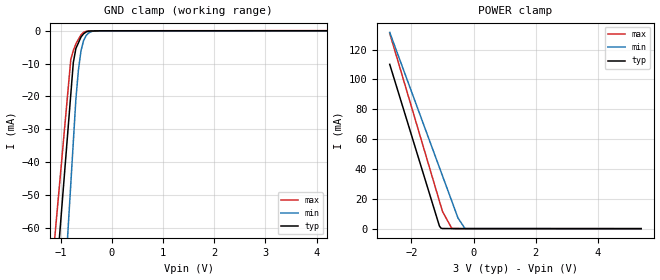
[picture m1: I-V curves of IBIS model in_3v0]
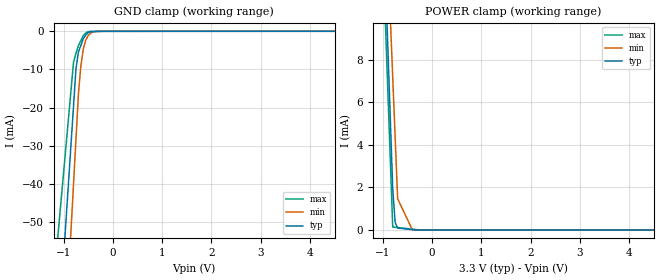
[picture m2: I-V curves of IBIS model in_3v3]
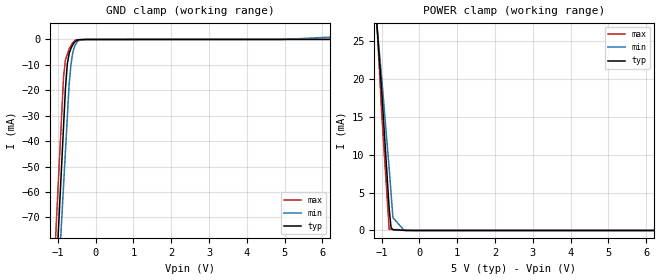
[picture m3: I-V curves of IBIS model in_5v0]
[IBIS Ver]   3.2
[Comment Char] |_char
[File Name]   tlv2553ipw.ibs
[File Rev]   3.0
[Source]
| This model file was created by Teraspeed Consulting Group LLC
| (http://www.teraspeed.com/).
[Date]   09-13-2007
[Notes]   Quality Check of this IBIS model: Model Passes IBIS Check
   Model parses into ICX IS. Simulation done with Hyperlynx.
   1. MIN TYP MAX information is based on Temprature and Voltage
   characteristics only.
[Disclaimer]
| This model is designed as an aid for customers of Texas Instruments.
| TI and its licensors and suppliers make no warranties, either expressed
| or implied, with respect to this  model, including the warranties of
| merchantability or fitness for a particular purpose.
| The model is provided solely on an "as is" basis. The entire risk as to
| its quality and performance is with the customer.
[Copyright]
| (C) Copyright 2008 Texas Instruments Incorporated. All rights reserved.
[Component] TLV2553IPW
[Manufacturer] TI
[Package]
| variable   typ   min   max
R_pkg  1.7363E-02  1.7363E-02  1.7363E-02
L_pkg  2.1878E-09  2.1878E-09  2.1878E-09
C_pkg  4.4649E-13  4.4649E-13  4.4649E-13
[Pin] signal_name  model_name  R_pin  L_pin C_pin
1   AIN0   term   1.97E-02  2.49E-09  5.07E-13
2   AIN1   term   1.89E-02  2.38E-09  4.85E-13
3   AIN2   term   1.80E-02  2.27E-09  4.64E-13
4   AIN3   term   1.72E-02  2.17E-09  4.42E-13
5   AIN4   term   1.64E-02  2.07E-09  4.22E-13
6   AIN5   term   1.56E-02  1.97E-09  4.02E-13
7   AIN6   term   1.49E-02  1.87E-09  3.82E-13
8   AIN7   term   1.49E-02  1.87E-09  3.82E-13
9   AIN8   term   1.56E-02  1.97E-09  4.02E-13
10   GND   GND   1.64E-02  2.07E-09  4.22E-13
11   AIN9   term   1.72E-02  2.17E-09  4.42E-13
12   AIN10   term   1.80E-02  2.27E-09  4.64E-13
13   REF-   term   1.89E-02  2.38E-09  4.85E-13
14   REF+   term   1.97E-02  2.49E-09  5.07E-13
15   _CS   input   1.97E-02  2.49E-09  5.07E-13
16   DATA_OUT  tri   1.89E-02  2.38E-09  4.85E-13
17   DATA_IN   input   1.80E-02  2.27E-09  4.64E-13
18   I/O_CLOCK input   1.72E-02  2.17E-09  4.42E-13
19   EOC   out   1.64E-02  2.07E-09  4.22E-13
20   VCC   POWER   1.56E-02  1.97E-09  4.02E-13
[Model Selector] input
in_3v0  3.0v input
in_3v3  3.3v input
in_5v0  5.0v input
[Model Selector] out
out_3v0  3.0v output
out_3v3  3.3v output
out_5v0  5.0v output
[Model Selector] tri
tri_3v0  3.0v 3-state
tri_3v3  3.3v 3-state
tri_5v0  5.0v 3-state
[Model] term
Model_type Terminator
C_comp  0pF 0pF 0pF
| variable typ   min   max
[Voltage Range]   5.00000V  4.50000V  5.50000V
[POWER Clamp Reference]  5.00000V  4.50000V  5.50000V
[GND Clamp Reference]   0.00000V  0.00000V  0.00000V
[Temperature Range]   25   105   -40
| Models and submodels in the file (10): in_3v0 (Input), in_3v3 (Input), in_5v0 (Input), out_3v0 (Output), out_3v3 (Output), out_5v0 (Output), tri_3v0 (3-state), tri_3v3 (3-state), tri_5v0 (3-state), term (Terminator)
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[Model] in_3v0
Model_type Input
Vinl = 600.000mV
Vinh = 2.10000V
C_comp 2.00000pF 2.00000pF 2.00000pF
| variable typ   min   max
[Voltage Range] 3.00000V 2.70000V 3.30000V
[POWER Clamp Reference] 3.00000V 2.70000V 3.30000V
[GND Clamp Reference] 0.00000V 0.00000V 0.00000V
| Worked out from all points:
|   GND clamp passes 1 mA (typ) near -0.55 V on its own axis
|   POWER clamp passes 1 mA (typ) near -1.07 V on its own axis
[GND Clamp]
-2.7V     -392.8mA   -540mA     -338.2mA
-800mV    -19.46mA   -46.76mA   -8.801mA
-750mV    -9.636mA   -33.78mA   -6.003mA
-700mV    -5.392mA   -20.8mA    -3.979mA
-650mV    -3.652mA   -11.85mA   -2.604mA
-600mV    -1.913mA   -6.079mA   -1.229mA
-550mV    -923.5uA   -2.99mA    -482.3uA
-500mV    -360.9uA   -1.469mA   -140.5uA
-450mV    -106uA     -655.1uA   -29.64uA
-350mV    -60.85uA   -75.9uA    -16.42uA
5.4V      3.964uA    7.545uA    59.3uA
[POWER Clamp]
-2.7V     110.1mA    131.5mA    130.8mA
-1.1V     1.801mA    41.03mA    18.52mA
-1.05V    353.6uA    38.2mA     15.01mA
-1V       103.6uA    35.37mA    11.5mA
-700mV    41.43uA    18.41mA    137.5uA
-500mV    0A         7.096mA    91.65uA
-275mV    0A         80.68uA    40.1uA
5.4V      0A         0A         0A
[Model] in_3v3
Model_type Input
Vinl = 600.000mV
Vinh = 2.10000V
C_comp 2.00000pF 2.00000pF 2.00000pF
| variable typ   min   max
[Voltage Range] 3.30000V 3.00000V 3.60000V
[POWER Clamp Reference] 3.30000V 3.00000V 3.60000V
[GND Clamp Reference] 0.00000V 0.00000V 0.00000V
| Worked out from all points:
|   GND clamp passes 1 mA (typ) near -0.55 V on its own axis
|   POWER clamp passes 1 mA (typ) near -0.77 V on its own axis
[GND Clamp]
-3.3V     -511.7mA   -633.6mA   -366.9mA
-800mV    -19.58mA   -40.06mA   -8.124mA
-750mV    -9.737mA   -28.19mA   -5.717mA
-700mV    -5.419mA   -16.32mA   -3.729mA
-650mV    -3.669mA   -8.949mA   -2.411mA
-600mV    -1.919mA   -4.533mA   -1.093mA
-550mV    -927.8uA   -2.25mA    -408.5uA
-500mV    -363.4uA   -1.085mA   -112.2uA
-450mV    -107.1uA   -455.5uA   -22.46uA
-400mV    -84.3uA    -156.3uA   -17.42uA
-175mV    -4.449uA   -2.224uA   618.4nA
6.6V      4.962uA    5.829uA    57.5uA
[POWER Clamp]
-3.3V     169.8mA    150.2mA    184.5mA
-1.15V    25.44mA    27.21mA    23.29mA
-1.1V     22.08mA    24.35mA    19.55mA
-800mV    1.939mA    7.185mA    140.4uA
-750mV    354.1uA    4.325mA    127.6uA
-700mV    90.64uA    1.465mA    114.8uA
-550mV    51.79uA    732.3uA    76.57uA
-400mV    12.95uA    0A         38.28uA
-350mV    0A         0A         25.52uA
-300mV    0A         0A         12.76uA
-150mV    0A         0A         0A
6.6V      0A         0A         0A
[Model] in_5v0
Model_type Input
Vinl = 800.000mV
Vinh = 2.00000V
C_comp 2.00000pF 2.00000pF 2.00000pF
| variable typ   min   max
[Voltage Range] 5.00000V 4.50000V 5.50000V
[POWER Clamp Reference] 5.00000V 4.50000V 5.50000V
[GND Clamp Reference] 0.00000V 0.00000V 0.00000V
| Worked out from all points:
|   GND clamp passes 1 mA (typ) near -0.55 V on its own axis
|   POWER clamp passes 1 mA (typ) near -0.76 V on its own axis
[GND Clamp]
-5V       -1.28A     -1.181A    -1.259A
-850mV    -34.55mA   -57.88mA   -15.05mA
-800mV    -19.55mA   -44.35mA   -8.058mA
-750mV    -9.671mA   -30.82mA   -5.87mA
-700mV    -5.406mA   -17.29mA   -3.681mA
-650mV    -3.391mA   -9.49mA    -2.376mA
-600mV    -1.914mA   -4.82mA    -1.07mA
-500mV    -361.2uA   -1.141mA   -108.6uA
-400mV    -82.86uA   -168.1uA   -66.09uA
-175mV    -818nA     -2.763uA   -1.276uA
4.95V     1.272uA    3.239uA    70.47uA
10V       3.332uA    3.628mA    141.2uA
[POWER Clamp]
-5V       295.8mA    242.3mA    392.6mA
-1.3V     39.41mA    36.99mA    44mA
-1V       18.62mA    20.34mA    15.73mA
-800mV    2.938mA    8.247mA    155.1uA
-750mV    385.4uA    4.974mA    143.2uA
-700mV    100.8uA    1.7mA      131.3uA
-400mV    14.4uA     0A         59.67uA
10V       0A         0A         0A
